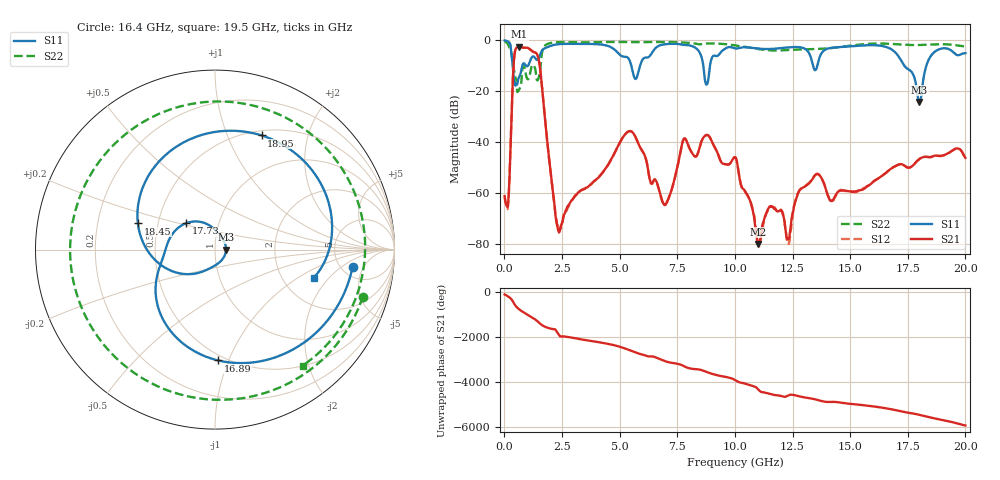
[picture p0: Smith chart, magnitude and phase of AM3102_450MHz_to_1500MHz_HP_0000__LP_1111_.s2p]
!Agilent Technologies,E8364B,MY43040894,A.07.50.67
!Agilent E8364B: A.07.50.67
!Date: Thursday, January 11, 2018 05:18:52
!Correction: S11(Full 2 Port(1,2))
!S21(Full 2 Port(1,2))
!S12(Full 2 Port(1,2))
!S22(Full 2 Port(1,2))
!S2P File: Measurements: S11, S21, S12, S22:
# Hz S  dB  R 50
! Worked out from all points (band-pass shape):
!   1601 points, 10 MHz to 20 GHz, reference 50 ohm
!   highest |S21| = -2.54 dB at 647.2 MHz (marker M1); lowest = -80.0 dB at 10.99 GHz (marker M2)
!   |S21| within 3 dB of the highest: 439.8 MHz to 1.421 GHz (981.5 MHz wide, 105 % of centre)
!   lowest |S11| = -24.2 dB at 18 GHz (marker M3), VSWR 1.13, Z = 56.5 - j0.0106 ohm
!   |S11| at or under -10 dB: 358.8 MHz to 777.6 MHz (418.8 MHz wide, 73.7 % of centre); 5.509 GHz to 5.887 GHz (377.7 MHz wide, 6.63 % of centre); 17.36 GHz to 18.3 GHz (949.3 MHz wide, 5.32 % of centre)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
!   |S22| runs from -20.3 to -0.5 dB; largest |S21 - S12| = 0.0034
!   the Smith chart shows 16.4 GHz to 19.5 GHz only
!   S11 on the Smith chart (normalised r, x): 16.4 GHz: 6.28, -3.05; 16.89 GHz: 0.46, -0.92; 17.73 GHz: 0.70, +0.22; 18.45 GHz: 0.38, +0.14; 18.95 GHz: 0.55, +1.34; 19.5 GHz: 2.95, -1.38
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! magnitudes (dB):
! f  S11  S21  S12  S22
! 10 MHz  0.0  -61.2  -61.4  -0.5
! 172.4 MHz  -0.6  -62.9  -63.4  -1.9
! 447.3 MHz  -16.7  -5.0  -5.0  -13.1
! 647.2 MHz  -14.3  -2.5  -2.5  -19.2
! 1.484 GHz  -7.1  -7.4  -7.4  -14.9
! 2.321 GHz  -1.5  -74.1  -72.9  -0.7
! 3.346 GHz  -1.4  -58.8  -58.7  -0.8
! 5.445 GHz  -8.1  -35.6  -35.6  -0.7
! 6.682 GHz  -2.2  -57.8  -57.8  -0.7
! 7.819 GHz  -1.8  -38.5  -38.5  -0.9
! 10.01 GHz  -3.2  -45.9  -45.9  -2.0
! 10.99 GHz  -3.2  -80.0  -79.1  -3.4
! 13.34 GHz  -8.2  -54.8  -54.7  -3.5
! 16.4 GHz  -2.2  -53.1  -53.0  -1.3
! 16.68 GHz  -3.0  -51.0  -51.0  -1.4
! 16.89 GHz  -4.2  -49.7  -49.7  -1.5
! 17.73 GHz  -13.3  -49.1  -49.2  -1.9
! 18 GHz  -24.2  -46.6  -46.6  -1.8
! 18.45 GHz  -6.9  -45.9  -45.9  -1.7
! 18.95 GHz  -3.3  -45.4  -45.4  -1.5
! 19.5 GHz  -4.9  -42.9  -42.9  -1.8
! 20 GHz  -5.0  -46.1  -46.2  -2.4
